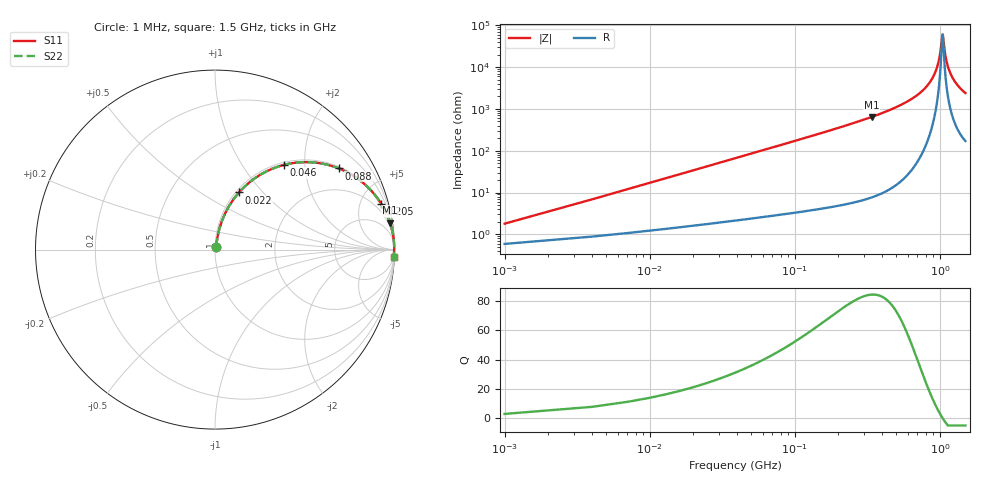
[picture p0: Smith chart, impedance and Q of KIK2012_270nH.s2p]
!version-2
!date-01.2022
!Series
# MHz S RI R 50
!Freq ReS11 ImS11 ReS21 ImS21 ReS12 ImS12 ReS22 ImS22
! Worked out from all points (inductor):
!   501 points, 1 MHz to 1.5 GHz, reference 50 ohm
!   read as one part in series: L = 270 nH near 7 MHz
!   highest Q = 84.4 at 340 MHz (marker M1), where L = 302 nH
!   self-resonance near 1.042 GHz
!   S11 on the Smith chart (normalised r, x): 1 MHz: 1.01, +0.03; 22 MHz: 1.03, +0.75; 46 MHz: 1.05, +1.56; 88 MHz: 1.06, +3.01; 205 MHz: 1.10, +7.23; 1.5 GHz: 4, -48
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1  0.00613 0.0168  0.9939 -0.0168  0.9939 -0.0168  0.00613 0.0168
10  0.0391 0.1611  0.9609 -0.1611  0.9609 -0.1611  0.0391 0.1611
16  0.0803 0.2461  0.9197 -0.2461  0.9197 -0.2461  0.0803 0.2461
22  0.1333 0.3183  0.8667 -0.3183  0.8667 -0.3183  0.1333 0.3183
46  0.3829 0.4717  0.6171 -0.4717  0.6171 -0.4717  0.3829 0.4717
88  0.6898 0.4524  0.3102 -0.4524  0.3102 -0.4524  0.6898 0.4524
136  0.8423 0.3563  0.1577 -0.3563  0.1577 -0.3563  0.8423 0.3563
205  0.926 0.255  0.074 -0.255  0.074 -0.255  0.926 0.255
253  0.9517 0.2081  0.0483 -0.2081  0.0483 -0.2081  0.9517 0.2081
340  0.9748 0.1508  0.0252 -0.1508  0.0252 -0.1508  0.9748 0.1508
502  0.9907 0.0893  0.0093 -0.0893  0.0093 -0.0893  0.9907 0.0893
751  0.9974 0.0378  0.00263 -0.0378  0.00263 -0.0378  0.9974 0.0378
913  0.9984 0.0152  0.00163 -0.0152  0.00163 -0.0152  0.9984 0.0152
964  0.9984 0.00905  0.00157 -0.00905  0.00157 -0.00905  0.9984 0.00905
1003  0.9984 0.00458  0.00159 -0.00458  0.00159 -0.00458  0.9984 0.00458
1036  0.9984 0.000944  0.00163 -0.000944  0.00163 -0.000944  0.9984 0.000944
1045  0.9983 -2.81e-05  0.00165 2.81e-05  0.00165 2.81e-05  0.9983 -2.81e-05
1087  0.9982 -0.00446  0.00177 0.00446  0.00177 0.00446  0.9982 -0.00446
1123  0.9981 -0.00812  0.0019 0.00812  0.0019 0.00812  0.9981 -0.00812
1177  0.9979 -0.0134  0.00215 0.0134  0.00215 0.0134  0.9979 -0.0134
1252  0.9974 -0.0204  0.00259 0.0204  0.00259 0.0204  0.9974 -0.0204
1500  0.9953 -0.0413  0.00468 0.0413  0.00468 0.0413  0.9953 -0.0413
